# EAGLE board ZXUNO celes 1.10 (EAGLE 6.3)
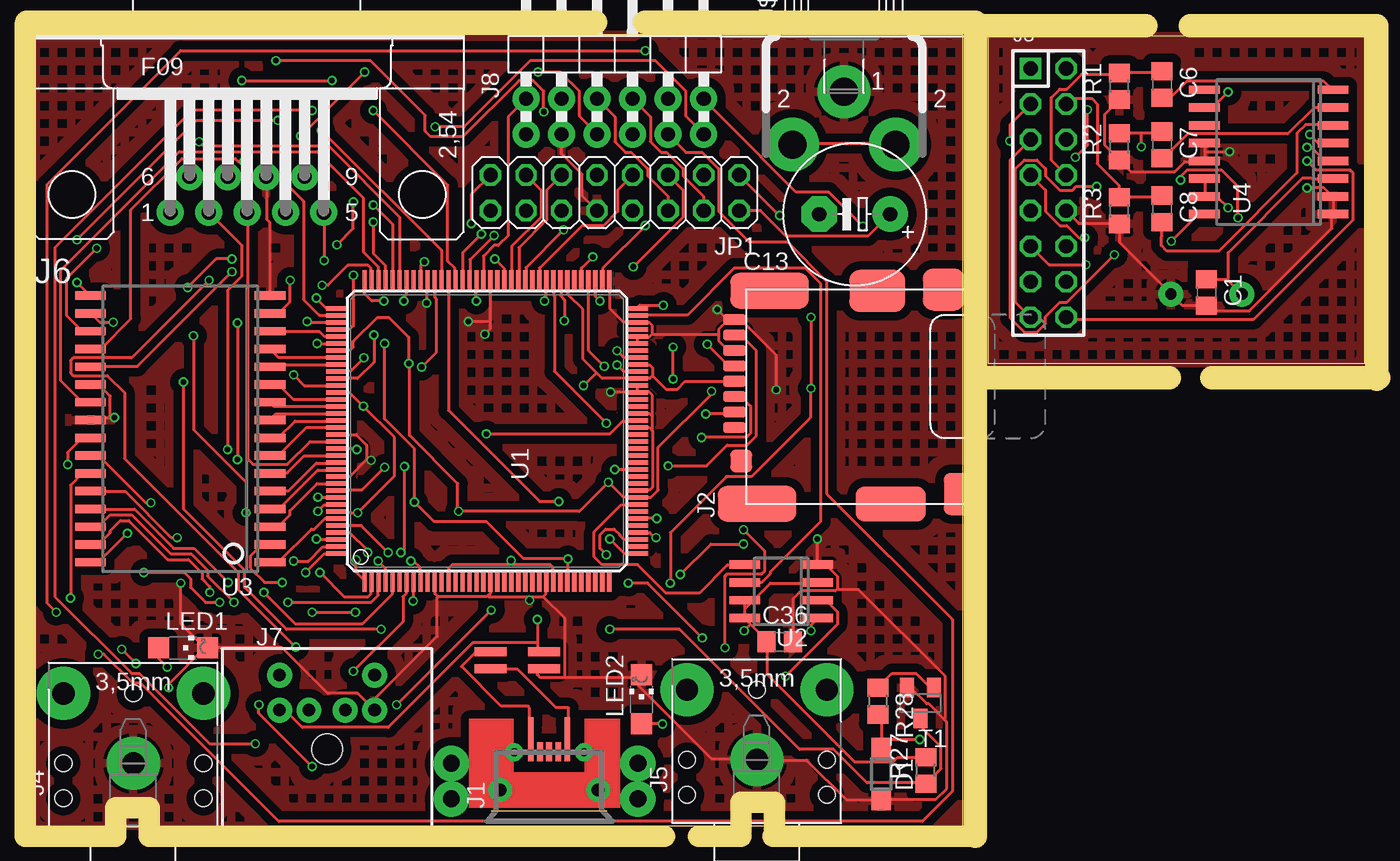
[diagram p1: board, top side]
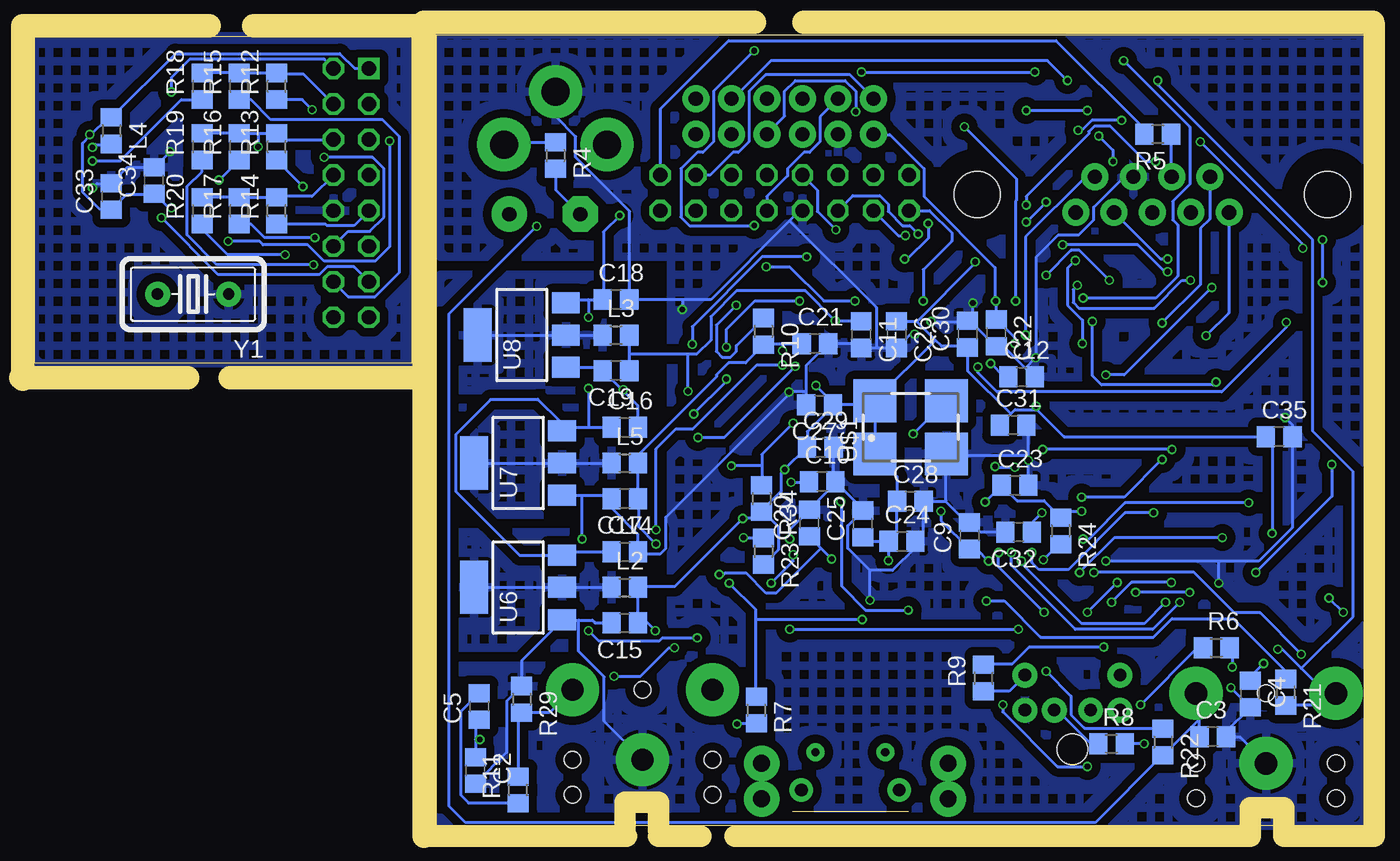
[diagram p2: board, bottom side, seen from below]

Size 95.05 x 56.49 mm. Coordinates in mm from the lower left corner, seen from the top.
Outline: 66.34,0 66.34,56.49 0,56.49 0,0 66.34,0
Outline: 68.12,56.39 68.12,33.02 95.05,33.02 95.05,56.39 68.12,56.39
Copper layers (1*16): Top 0.035mm / dielectric 1.5mm / Bottom 0.035mm
Design rules "default *": minimum track width 8mil, minimum drill 16mil, track to track 8mil, track to pad 8mil, pad to pad 8mil, via to via 10mil, smd to smd 8mil, copper to edge 0mil, drill to drill 10mil, minimum pad ring 5mil, minimum via ring 5mil, stop-mask expansion 4mil, vias tented up to drill 0mil, thermal gap 10mil
Net classes: 1 alimentacion: width 0.203 mm, drill 0.203 mm, clearance 0.203 mm
Milling: 19 lines

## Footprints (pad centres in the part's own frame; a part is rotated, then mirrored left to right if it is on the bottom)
C0805 = smd 1.3 x 1.5: 1 -0.95,0; 2 0.95,0
E5-10,5 = drill 1.016 pad 2.54: + -2.54,0 | drill 1.016 pad 2.54 octagon: - 2.54,0
SOD123 = smd 1.4 x 1.4: A 1.9,0; C -1.9,0
MICRO_USB = smd 1.35 x 0.4: 1 2.73,1.3; 2 2.73,0.65; 3 2.73,0; 4 2.73,-0.65; 5 2.73,-1.3; 6 4,1.3; 10 4,-1.3; 11 4.508,1.3; 13 4.508,-1.3 | drill 0.6 pad 1.27: P$1 2.7,2.5; P$2 2.7,-2.5 | drill 0.9 pad 1.676: P$3 0,3.5; P$4 0,-3.5 | drill 1.2 pad 2.54: P$5 -0.635,6.985; P$6 1.905,6.985; P$7 -0.635,-6.35; P$8 1.905,-6.35
MICRO_SD_CONNECTOR = smd 0.8 x 1.6: 1 -2.03,8.2; 2 -0.93,8.2; 3 0.17,8.2; 4 1.27,8.2; 5 2.37,8.2; 6 3.47,8.2; 7 4.57,8.2; 8 5.67,8.2 | smd 2.54 x 5.588: 9 7.735,5.7; 14 -7.49,6.6 | smd 3 x 4: 10 7.735,-2 | smd 3 x 3: 11 7.81,-6.75 | smd 3 x 2: 12 -6.79,-7.75 | smd 2.5 x 5: 13 -7.49,-2.95 | smd 1.6 x 1.55: 15 -4.43,7.725
DIL-100-2X08 = drill 1.016 square: 1 -8.89,-1.27 | drill 1.016 octagon: 2 -8.89,1.27; 3 -6.35,-1.27; 4 -6.35,1.27; 5 -3.81,-1.27; 6 -3.81,1.27; 7 -1.27,-1.27; 8 -1.27,1.27; 9 1.27,-1.27; 10 1.27,1.27; 11 3.81,-1.27; 12 3.81,1.27; 13 6.35,-1.27; 14 6.35,1.27; 15 8.89,-1.27; 16 8.89,1.27
STX = drill 1.6 pad 3.81: P$1 -0.762,-0.127; P$2 4.242,-5.131; P$3 4.242,4.877 | hole 1.2: -3.251,4.877; -0.762,4.877; -0.762,-5.131; -3.251,-5.131; 4.242,-0.127
F09H = drill 1.016 pad 1.93: 1 -5.486,-1.27; 2 -2.743,-1.27; 3 0,-1.27; 4 2.743,-1.27; 5 5.486,-1.27; 6 -4.115,1.27; 7 -1.372,1.27; 8 1.372,1.27; 9 4.115,1.27 | hole 3.302: -12.522,0; 12.522,0
MDIN06SS = drill 0.9 pad 1.778: 1 1.3,8.5; 2 -1.3,8.5; 3 3.4,8.5; 4 -3.4,8.5; 5 3.4,11; 6 -3.4,11 | hole 2.2: 0,5.716
2X06/90 = drill 1.016 pad 1.93: 1 -6.35,-6.35; 2 -6.35,-3.81; 3 -3.81,-6.35; 4 -3.81,-3.81; 5 -1.27,-6.35; 6 -1.27,-3.81; 7 1.27,-6.35; 8 1.27,-3.81; 9 3.81,-6.35; 10 3.81,-3.81; 11 6.35,-6.35; 12 6.35,-3.81
2X08 = drill 1.016 octagon: 1 -8.89,-1.27; 2 -8.89,1.27; 3 -6.35,-1.27; 4 -6.35,1.27; 5 -3.81,-1.27; 6 -3.81,1.27; 7 -1.27,-1.27; 8 -1.27,1.27; 9 1.27,-1.27; 10 1.27,1.27; 11 3.81,-1.27; 12 3.81,1.27; 13 6.35,-1.27; 14 6.35,1.27; 15 8.89,-1.27; 16 8.89,1.27
CHOKE_COMM = smd 1.27 x 0.635: P$1 -1.4,0.6; P$2 -1.4,-0.6; P$3 1.4,-0.6; P$4 1.4,0.6; P$5 -2.416,0.6; P$6 -2.416,-0.6; P$7 2.416,0.6; P$8 2.416,-0.6
0805 = smd 1.3 x 1.5: 1 -0.95,0; 2 0.95,0
CHIPLED_1206 = smd 1.5 x 1.5: A 0,-1.75; C 0,1.75
R0805 = smd 1.3 x 1.5: 1 -0.95,0; 2 0.95,0
SOT23 = smd 1 x 1.4: 1 -0.95,-1.1; 2 0.95,-1.1; 3 0,1.1
TQ144 = smd 1.6 x 0.3: P1 -10.7,8.75; P2 -10.7,8.25; P3 -10.7,7.75; P4 -10.7,7.25; P5 -10.7,6.75; P6 -10.7,6.25; P7 -10.7,5.75; P8 -10.7,5.25; P9 -10.7,4.75; P10 -10.7,4.25; P11 -10.7,3.75; P12 -10.7,3.25; P13 -10.7,2.75; P14 -10.7,2.25; P15 -10.7,1.75; P16 -10.7,1.25; P17 -10.7,0.75; P18 -10.7,0.25; P19 -10.7,-0.25; P20 -10.7,-0.75; P21 -10.7,-1.25; P22 -10.7,-1.75; P23 -10.7,-2.25; P24 -10.7,-2.75; P25 -10.7,-3.25; P26 -10.7,-3.75; P27 -10.7,-4.25; P28 -10.7,-4.75; P29 -10.7,-5.25; P30 -10.7,-5.75; P31 -10.7,-6.25; P32 -10.7,-6.75; P33 -10.7,-7.25; P34 -10.7,-7.75; P35 -10.7,-8.25; P36 -10.7,-8.75; P73 10.7,-8.75; P74 10.7,-8.25; P75 10.7,-7.75; P76 10.7,-7.25; P77 10.7,-6.75; P78 10.7,-6.25; P79 10.7,-5.75; P80 10.7,-5.25; P81 10.7,-4.75; P82 10.7,-4.25; P83 10.7,-3.75; P84 10.7,-3.25; P85 10.7,-2.75; P86 10.7,-2.25; P87 10.7,-1.75; P88 10.7,-1.25; P89 10.7,-0.75; P90 10.7,-0.25; P91 10.7,0.25; P92 10.7,0.75; P93 10.7,1.25; P94 10.7,1.75; P95 10.7,2.25; P96 10.7,2.75; P97 10.7,3.25; P98 10.7,3.75; P99 10.7,4.25; P100 10.7,4.75; P101 10.7,5.25; P102 10.7,5.75; P103 10.7,6.25; P104 10.7,6.75; P105 10.7,7.25; P106 10.7,7.75; P107 10.7,8.25; P108 10.7,8.75 | smd 0.3 x 1.6: P37 -8.75,-10.7; P38 -8.25,-10.7; P39 -7.75,-10.7; P40 -7.25,-10.7; P41 -6.75,-10.7; P42 -6.25,-10.7; P43 -5.75,-10.7; P44 -5.25,-10.7; P45 -4.75,-10.7; P46 -4.25,-10.7; P47 -3.75,-10.7; P48 -3.25,-10.7; P49 -2.75,-10.7; P50 -2.25,-10.7; P51 -1.75,-10.7; P52 -1.25,-10.7; P53 -0.75,-10.7; P54 -0.25,-10.7; P55 0.25,-10.7; P56 0.75,-10.7; P57 1.25,-10.7; P58 1.75,-10.7; P59 2.25,-10.7; P60 2.75,-10.7; P61 3.25,-10.7; P62 3.75,-10.7; P63 4.25,-10.7; P64 4.75,-10.7; P65 5.25,-10.7; P66 5.75,-10.7; P67 6.25,-10.7; P68 6.75,-10.7; P69 7.25,-10.7; P70 7.75,-10.7; P71 8.25,-10.7; P72 8.75,-10.7; P109 8.75,10.7; P110 8.25,10.7; P111 7.75,10.7; P112 7.25,10.7; P113 6.75,10.7; P114 6.25,10.7; P115 5.75,10.7; P116 5.25,10.7; P117 4.75,10.7; P118 4.25,10.7; P119 3.75,10.7; P120 3.25,10.7; P121 2.75,10.7; P122 2.25,10.7; P123 1.75,10.7; P124 1.25,10.7; P125 0.75,10.7; P126 0.25,10.7; P127 -0.25,10.7; P128 -0.75,10.7; P129 -1.25,10.7; P130 -1.75,10.7; P131 -2.25,10.7; P132 -2.75,10.7; P133 -3.25,10.7; P134 -3.75,10.7; P135 -4.25,10.7; P136 -4.75,10.7; P137 -5.25,10.7; P138 -5.75,10.7; P139 -6.25,10.7; P140 -6.75,10.7; P141 -7.25,10.7; P142 -7.75,10.7; P143 -8.25,10.7; P144 -8.75,10.7
SO-08 = smd 0.6 x 2.2: 1 -1.905,-2.6; 2 -0.635,-2.6; 3 0.635,-2.6; 4 1.905,-2.6; 5 1.905,2.6; 6 0.635,2.6; 7 -0.635,2.6; 8 -1.905,2.6
SOIC32 = smd 0.6 x 2.2: 1 -9.525,-6.416; 2 -8.255,-6.416; 3 -6.985,-6.416; 4 -5.715,-6.416; 5 -4.445,-6.416; 6 -3.175,-6.416; 7 -1.905,-6.416; 8 -0.635,-6.416; 9 0.635,-6.416; 10 1.905,-6.416; 11 3.175,-6.416; 12 4.445,-6.416; 13 5.715,-6.416; 14 6.985,-6.416; 15 8.255,-6.416; 16 9.525,-6.416; 17 9.525,6.416; 18 8.255,6.416; 19 6.985,6.416; 20 5.715,6.416; 21 4.445,6.416; 22 3.175,6.416; 23 1.905,6.416; 24 0.635,6.416; 25 -0.635,6.416; 26 -1.905,6.416; 27 -3.175,6.416; 28 -4.445,6.416; 29 -5.715,6.416; 30 -6.985,6.416; 31 -8.255,6.416; 32 -9.525,6.416
SO16W = smd 0.6 x 2.2: 1 -4.445,-4.6; 2 -3.175,-4.6; 3 -1.905,-4.6; 4 -0.635,-4.6; 5 0.635,-4.6; 6 1.905,-4.6; 7 3.175,-4.6; 8 4.445,-4.6; 9 4.445,4.6; 10 3.175,4.6; 11 1.905,4.6; 12 0.635,4.6; 13 -0.635,4.6; 14 -1.905,4.6; 15 -3.175,4.6; 16 -4.445,4.6
SOT223 = smd 1.5 x 2: 1 -2.3,-3.15; 2 0,-3.15; 3 2.3,-3.15 | smd 3.8 x 2: 4 0,3.15
SM77H = smd 3.048 x 3.048: 1 -2.55,-1.9; 2 2.55,-1.9; 3 2.55,1.9; 4 -2.55,1.9
RCA_PACK = drill 2 pad 3.81: 1 0,-3.945; 2 3.688,-7.72; 2@1 -3.688,-7.72
HC18U-V = drill 0.813 pad 1.778: 1 -2.54,0; 2 2.54,0

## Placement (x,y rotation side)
C1  8pF  [C0805]  83.74,38.1 270 top
C2  10nF  [C0805]  63.55,3.94 270 bottom
C3  10nF  [C0805]  10.85,6.35 0 bottom
C4  10nF  [C0805]  8.18,9.4 270 bottom
C5  100nF  [C0805]  63.3,8.51 90 bottom
C6  100nF  [C0805]  80.57,52.96 270 top
C7  100nF  [C0805]  80.57,48.64 270 top
C8  100nF  [C0805]  80.57,44.07 270 top
C9  100nF  [C0805]  28.24,20.71 90 bottom
C10  100nF  [C0805]  38.78,24.57 0 bottom
C11  100nF  [C0805]  35.98,35.08 270 bottom
C12  100nF  [C0805]  24.52,32.07 0 bottom
C13  220uF  [E5-10,5]  58.6,43.69 180 top
C14  1uF  [C0805]  52.88,19.56 0 bottom
C15  1uF  [C0805]  52.88,14.48 180 bottom
C16  1uF  [C0805]  52.88,28.45 0 bottom
C17  1uF  [C0805]  52.88,23.37 180 bottom
C18  1uF  [C0805]  53.52,37.59 0 bottom
C19  1uF  [C0805]  53.52,32.51 180 bottom
C20  100nF  [C0805]  39.68,21.62 90 bottom
C21  100nF  [C0805]  39.28,34.44 0 bottom
C22  100nF  [C0805]  26.33,35.21 270 bottom
C23  100nF  [C0805]  24.99,24.3 0 bottom
C24  100nF  [C0805]  33.06,20.31 0 bottom
C25  100nF  [C0805]  35.87,21.56 90 bottom
C26  100nF  [C0805]  33.46,35.08 270 bottom
C27  100nF  [C0805]  38.96,30.07 180 bottom
C28  100nF  [C0805]  32.46,23.18 0 bottom
C29  100nF  [C0805]  38.9,27.02 0 bottom
C30  100nF  [C0805]  28.38,35.12 90 bottom
C31  100nF  [C0805]  25.12,28.62 0 bottom
C32  100nF  [C0805]  24.73,20.96 180 bottom
C33  100nF  [C0805]  89.59,44.96 90 bottom
C34  10uF  [C0805]  86.54,46.1 90 bottom
C35  100nF  [C0805]  6.1,27.79 0 bottom
C36  100nF  [C0805]  53.24,13.13 0 top
D1  [SOD123]  60.5,3.68 270 top
J1  CON_MICRO_USB  [MICRO_USB]  36.75,2.54 90 top
J2  MICROSD_SPI_MODE  [MICRO_SD_CONNECTOR]  58.22,30.48 90 top
J3  J-16-100-2X08  [DIL-100-2X08]  72.44,45.21 270 top
J4  JACK_STEREO  [STX]  6.91,5.21 90 top
J5  JACK_STEREO  [STX]  51.49,5.46 90 top
J6  [F09H]  15.16,45.09 0 top
J7  [MDIN06SS]  20.88,-0.25 0 top
J8  JTAG_RGB  [2X06/90]  41.45,55.75 0 top
JP1  [2X08]  41.45,45.21 180 top
L1  BOBINA_VCC_ZXUNO  [CHOKE_COMM]  34.47,11.81 0 top
L2  FERRITE  [0805]  52.88,17.02 0 bottom
L3  FERRITE  [0805]  53.52,35.05 0 bottom
L4  FERRITE  [0805]  89.59,49.66 270 bottom
L5  FERRITE  [0805]  52.88,25.91 0 bottom
LED1  [CHIPLED_1206]  10.59,12.7 270 top
LED2  [CHIPLED_1206]  43.36,9.02 0 top
R1  75  [R0805]  77.52,52.83 90 top
R2  75  [R0805]  77.52,48.51 90 top
R3  75  [R0805]  77.52,43.94 90 top
R4  75  [R0805]  57.84,47.88 270 bottom
R5  270  [R0805]  14.78,49.4 180 bottom
R6  100  [R0805]  10.59,12.7 0 bottom
R7  220  [R0805]  43.48,8.26 270 bottom
R8  270  [R0805]  18.08,5.84 0 bottom
R9  270  [R0805]  27.23,10.54 90 bottom
R10  330  [R0805]  42.97,35.32 270 bottom
R11  470  [R0805]  60.5,2.54 90 bottom
R12  470  [R0805]  77.78,52.83 90 bottom
R13  470  [R0805]  77.78,48.51 90 bottom
R14  470  [R0805]  77.78,43.94 90 bottom
R15  1K  [R0805]  80.44,52.83 90 bottom
R16  1K  [R0805]  80.44,48.51 90 bottom
R17  1K  [R0805]  80.44,43.94 90 bottom
R18  2K  [R0805]  83.11,52.83 90 bottom
R19  2K  [R0805]  83.11,48.51 90 bottom
R20  2K  [R0805]  83.11,43.94 90 bottom
R21  3K9  [R0805]  5.64,9.53 270 bottom
R22  3K9  [R0805]  14.4,5.97 270 bottom
R23  4K7  [R0805]  42.97,19.6 270 bottom
R24  4K7  [R0805]  21.72,21.05 270 bottom
R27  1OK  [R0805]  63.68,3.94 90 top
R28  10K  [R0805]  60.25,8.89 270 top
R29  10K  [R0805]  60.25,9.02 270 bottom
R34  10K  [R0805]  43.1,23.37 270 bottom
T1  BC846  [SOT23]  63.3,8.76 180 top
U1  XC3S250ETQ144  [TQ144]  32.31,28.19 90 top
U2  W25X40BV  [SO-08]  53.35,16.74 90 top
U3  CY62148EV30  [SOIC32]  10.39,28.34 90 top
U4  AD724JR  [SO16W]  88.19,48.13 90 top
U6  LD117AS33TR  [SOT223]  60.5,17.02 90 bottom
U7  LD117AS25TR  [SOT223]  60.5,25.91 90 bottom
U8  LD117AS12TR  [SOT223]  60.25,35.05 90 bottom
U$1  SIT1602AC-83  [SM77H]  32.44,28.46 0 bottom
U$3  RCA_VIDEO  [RCA_PACK]  57.84,56.39 0 top
Y1  4.43M/3.58M  [HC18U-V]  83.74,37.97 180 bottom

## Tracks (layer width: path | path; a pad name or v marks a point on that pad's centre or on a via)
1.2V  (via drill 0.41)
  Top 0.203: v37.85,36.07 37.85,37.59 37.59,37.85 37.59,38.86 U1.P80 | U1.P115 21.64,33.98 22.55,33.98 22.76,34.19 22.76,34.59 24.49,36.32 25.3,36.32 26.72,34.9 v26.72,33.02 26.77,32.97 26.77,27.89 30.23,24.43 30.23,22.5 v30.28,22.45 38.91,22.45 v41,24.54 42.06,23.47 42.98,23.47 U1.P45 43.08,23.47 44.04,23.47 44.55,23.98 44.55,27.03 48.36,30.84 v48.36,31.04 | v26.87,18.9 27.08,18.9 27.53,18.44 27.53,17.53 U1.P9
  Bottom 0.203: 52.58,33.68 L3.2 | 52.58,33.68 C19.1 | C11.1 36.02,36.07 v37.85,36.07 39.98,38.2 44.91,38.2 46.74,36.37 46.74,34.7 47.75,33.68 48.36,33.68 | 48.36,33.68 52.58,33.68 | v26.72,33.02 25.81,32.11 25.5,32.11 C12.1 | v26.87,18.9 27.69,19.71 28.19,19.71 C9.1 28.3,19.81 30.28,21.79 v30.28,22.45 | v41,24.54 39.78,24.54 C10.1 | v48.36,31.04 48.36,33.68
2.5V  (via drill 0.41)
  Top 0.203: v26.36,37.49 26.36,37.8 26.52,37.95 26.52,38.86 U1.P102 | v41.61,33.93 42.06,33.48 42.98,33.48 U1.P65 | U1.P30 38.1,17.53 v38.1,19.05 38.05,19.1 34.9,19.1 32.26,21.74 28.5,21.74 v27.13,23.11 27.13,26.92 24.99,29.06 v24.99,34.44 | v20.22,22.45 20.68,22.91 21.59,22.91 U1.P137 | v50.65,20.12 48.31,20.12 v46.13,17.93
  Bottom 0.203: J8.1 35.1,49.38 33.94,49.38 31.5,46.94 31.5,44.96 26.42,39.88 26.42,37.54 v26.36,37.49 26.36,36.17 C22.1 26.26,36.12 24.99,34.85 v24.99,34.44 | 41.61,34.39 40.34,34.39 40.29,34.44 C21.1 | 41.61,34.39 42.93,34.39 R10.2 43.03,34.29 44.25,33.07 45.47,33.07 46.33,32.21 46.33,32.05 51.87,26.52 51.87,25.96 L5.2 51.97,25.91 51.97,23.37 C17.1 51.87,23.32 51.87,21.34 v50.65,20.12 | 41.61,34.39 v41.61,33.93 | v38.1,19.05 38.86,19.81 | 38.86,19.81 39.68,20.62 C20.1 | v20.22,22.45 22.05,22.45 R24.1 21.74,22.05 22.91,23.22 24.84,23.22 25.91,24.28 C23.1 26.01,24.23 v27.13,23.11 | v46.13,17.93 45.82,17.93 45.72,18.03 44.2,18.03 42.77,16.61 42.06,16.61 38.86,19.81
3.3V  (via drill 0.41)
  Top 0.203: U1.P138 21.64,22.4 22.55,22.4 22.61,22.35 v23.06,22.35 25.7,24.99 25.7,27.74 v23.47,29.97 22.5,30.94 21.64,30.94 U1.P121 | v27.84,40.28 27.58,40.03 27.58,38.91 U1.P100 | v6.6,20.88 4.57,18.85 4.01,18.85 U3.32 | 51.16,14.38 50.75,14.78 U2.8 50.75,14.88 50.75,15.54 | 51.16,14.38 52.27,13.26 52.27,13.16 C36.1 52.32,13.06 52.32,10.82 58.57,4.57 61.37,4.57 61.67,4.88 63.65,4.88 R27.2 | 50.75,15.54 50.75,16.05 U2.7 | U2.3 55.93,17.32 52.58,17.32 50.8,15.54 50.75,15.54 | 44.15,32.16 43.94,31.95 43.03,31.95 U1.P62 42.93,31.95 40.54,31.95 40.13,32.36 | 44.15,32.16 44.15,32.72 43.94,32.92 43.03,32.92 U1.P64 | 40.13,32.36 39.17,33.33 39.17,36.88 38.1,37.95 38.1,38.86 U1.P79 | J2.4 46.48,31.75 45.92,31.19 45.11,31.19 44.15,32.16 | v44.45,21.95 43.03,21.95 U1.P42 | 34.04,18.64 36.83,18.64 37.03,18.44 37.03,17.53 U1.P28 | 34.04,18.64 29.82,18.64 29.57,18.39 29.57,17.53 U1.P13 | v41.45,25.45 42.98,25.45 U1.P49 | v34.04,18.95 34.04,18.64 | v39.22,31.45 40.13,32.36 | v50.7,13.92 51.16,14.38
  Bottom 0.203: v23.06,22.35 23.77,21.64 23.77,20.98 C32.1 | 23.42,29.72 21.49,27.79 C35.1 6.96,27.74 6.6,27.38 v6.6,20.88 | 23.42,29.72 24.99,29.72 25.3,29.41 | 25.3,29.41 26.06,28.65 C31.1 | 25.3,29.41 28.35,32.46 28.35,34.14 C30.1 28.45,34.24 30.23,34.24 30.68,34.7 | 32,36.02 33.43,36.02 C26.1 | 30.68,34.7 32,36.02 | v27.84,40.28 27.84,40.18 32,36.02 | v23.47,29.97 23.47,29.77 23.42,29.72 | R23.2 42.93,18.69 41.91,19.71 41.91,21.34 42.98,22.4 43.08,22.4 R34.2 | R34.2 42.62,21.95 v44.45,21.95 49.33,17.07 51.87,17.07 L2.2 51.97,17.02 51.97,14.48 C15.1 51.92,15.14 v50.7,13.92 | C24.1 34.04,20.32 35.61,20.32 35.87,20.57 C25.1 | C24.1 33.94,20.37 33.43,20.88 33.43,23.16 C28.1 33.43,23.27 33.43,24.94 34.95,26.47 U$1.1 35,30.23 U$1.4 | C27.1 38,30.07 35.26,30.07 35,30.33 U$1.4 | C27.1 38,29.97 39.83,28.14 39.83,27.03 C29.1 39.93,26.98 v41.45,25.45 41.71,25.2 41.71,23.88 42.93,22.66 42.93,22.45 R34.2 | v34.04,18.95 34.04,20.22 C24.1 | v39.22,31.45 37.9,30.12 C27.1 | 30.68,34.7 34.95,30.43 U$1.4
5V  (via drill 0.41)
  Top 0.203: JP1.1 v53.24,43.59 | v55.47,36.32 v55.47,31.24 55.42,31.19 55.42,29.16 51.21,24.94 49.43,24.94 45.41,20.93 v45.41,17.32 | v35.92,14.73 35.92,13.06 | 35.92,13.06 35.92,12.45 L1.P$4 | J7.4 17.53,8.23 17.88,8.23 19.1,7.01 25.25,7.01 31.29,13.06 35.92,13.06
  Bottom 0.203: C14.1 57.1,19.56 57.3,19.36 U6.3 57.46,19.3 60.4,19.3 64.97,23.88 64.97,27.94 62.48,30.43 59.18,30.43 59.11,30.48 57.46,28.83 57.46,28.19 U7.3 57.3,28.25 57.1,28.45 55.47,28.45 | 55.47,28.45 C16.1 | 55.47,37.59 56.84,37.59 57.05,37.39 U8.3 | 55.47,37.59 C18.1 54.41,37.64 54.41,42.42 v53.24,43.59 | JP1.1 50.34,51.21 45.47,56.08 22.05,56.08 15.75,49.78 15.75,49.43 R5.2 | v55.47,31.24 55.47,28.45 | 55.47,37.59 v55.47,36.32 | 43.54,14.73 43.54,15.44 v45.41,17.32 | 43.54,14.73 43.54,9.3 R7.1 | 43.54,14.73 v35.92,14.73
5V_  (via drill 0.41)
  Top 0.203: U4.14 83.62,46.23 83.62,44.96 U4.15 83.67,44.91 84.53,44.91 v85.29,44.15 | U4.5 91.75,48.77 v91.14,49.38
  Bottom 0.203: 91.09,49.33 91.64,48.77 91.64,45.26 90.42,44.04 89.66,44.04 C33.1 89.56,44.04 88.49,45.11 86.56,45.11 C34.1 86.46,45.11 85.5,44.15 v85.29,44.15 | 91.09,49.33 89.81,50.6 89.61,50.6 L4.1 89.51,50.65 84.99,55.17 73.25,55.17 72.19,54.1 J3.1 | v91.14,49.38 91.09,49.33
B
  Top 0.203: JP1.4 47.8,44.96 46.33,46.43 46.33,46.94 45.16,48.11 44.76,48.11 43.99,48.87 43.99,50.65 42.72,51.92 J8.8
B0  (via drill 0.41)
  Top 0.203: v31.55,37.49 31.55,38.86 U1.P92
  Bottom 0.203: v31.55,37.49 31.55,39.73 29.51,41.76 29.51,42.37 31.09,43.94 JP1.16
B0_  (via drill 0.41)
  Top 0.203: v90.93,47.5 91.59,46.84 94.03,46.84 94.23,46.63 94.23,43.28 87.12,36.17 73.86,36.17 J3.16
  Bottom 0.203: v90.93,47.5 88.95,47.5 84.58,51.87 83.11,51.87 R18.1
B1  (via drill 0.41)
  Top 0.203: v32.82,42.16 31.09,40.44 31.09,38.91 U1.P93
  Bottom 0.203: v32.82,42.16 33.33,42.16 JP1.14
B1_
  Bottom 0.203: J3.14 72.64,37.8 70.71,37.8 68.99,39.52 68.99,49.23 70.21,50.44 78.18,50.44 79.6,51.87 80.42,51.87 R15.1
B2  (via drill 0.41)
  Top 0.203: v31.9,42.27 30.58,40.95 30.58,38.91 U1.P94
  Bottom 0.203: v31.9,42.27 32.51,42.88 33.02,42.88 34.04,43.89 34.04,44.4 34.65,45.01 36.58,45.01 JP1.12
B2_  (via drill 0.41)
  Top 0.203: v75.23,51.16 75.23,48.62 v74.37,47.75
  Bottom 0.203: v75.23,51.16 75.95,51.87 77.78,51.87 R12.1 | v74.37,47.75 70.92,47.75 70.1,46.94 70.1,43.48 71.12,42.47 72.64,42.47 J3.12
B_
  Top 0.203: C8.1 80.47,44.91 77.52,44.91 R3.2 77.47,44.96 77.47,45.77 75.95,47.3 75.95,51.56 75.54,51.97 74.12,51.97 J3.4
  Bottom 0.203: R18.2 83.11,53.8 80.52,53.8 R15.2 80.42,53.8 77.78,53.8 R12.2 77.72,53.7 75.84,53.7 J3.4
CLK  (via drill 0.41)
  Top 0.203: v32.26,27.99 41.1,27.99 42.01,28.91 42.98,28.91 U1.P56
  Bottom 0.203: v32.26,27.99 29.92,30.33 U$1.3
CMPS
  Top 0.203: JP1.2 51.87,43.94 53.7,42.11 59.54,42.11 61.11,43.69 C13.+
CMPS_  (via drill 0.41)
  Top 0.203: U4.10 84.18,51.31 v85.29,52.43
  Bottom 0.203: v85.29,52.43 85.29,53.44 83.97,54.76 74.37,54.76 J3.2
CSYNC
  Top 0.203: U1.P91 32.05,38.91 32.05,40.69 32.82,41.45 33.12,41.45 33.83,42.16 33.83,50.65 35.1,51.92 J8.2
  Bottom 0.203: JP1.3 46.79,46.48 45.16,48.11 44.76,48.11 43.99,48.87 43.99,52.48 42.83,53.65 36.78,53.65 35.1,51.97 J8.2
CSYNC_  (via drill 0.41)
  Top 0.203: U4.16 83.16,43.69 v81.23,41.76 | v69.7,48.92 69.7,50.09 J3.3
  Bottom 0.203: v81.23,41.76 78.99,41.76 78.74,41.5 75.54,41.5 74.37,40.34 70.71,40.34 69.7,41.35 v69.7,48.92
EAR  (via drill 0.41)
  Top 0.203: T1.3 63.3,7.11 64.77,5.64 64.77,4.06 63.7,3 R27.1 63.6,3.05 59.49,3.05 57.1,5.44 54.66,5.44 46.08,14.02 v41.1,14.02 | v19.46,36.02 19.51,35.97 21.59,35.97 U1.P111 | v10.62,31.7 10.62,22.61 14.99,18.24 14.99,17.02 17.98,14.02 v24.74,14.02
  Bottom 0.203: v19.46,36.02 19.46,32.16 18.8,31.5 10.82,31.5 v10.62,31.7 | v41.1,14.02 v24.74,14.02
FLASH_CS  (via drill 0.41)
  Top 0.203: v40.84,19.36 40.39,19.81 40.39,20.78 40.79,21.18 41.4,21.18 41.81,20.78 41.81,20.73 42.06,20.47 42.98,20.47 U1.P39 | v42.42,17.32 43.79,17.32 v47.7,13.41 | v55.47,13.92 55.47,14.33 55.93,14.78 U2.1
  Bottom 0.203: v40.84,19.36 40.84,18.9 v42.42,17.32 | v47.7,13.41 50.19,13.41 50.39,13.21 54.76,13.21 v55.47,13.92
FLASH_MISO  (via drill 0.41)
  Top 0.203: v41.61,32.92 42.06,32.46 42.98,32.46 U1.P63 | v50.65,21.13 52.17,19.61 52.17,18.19 51.97,17.98 49.48,17.98 49.33,17.83 v49.33,12.7 | v53.65,10.67 57.35,14.38 57.35,15.29 56.59,16.05 55.98,16.05 U2.2
  Bottom 0.203: v41.61,32.92 43.43,32.92 48.01,28.35 49.23,28.35 50.65,26.92 v50.65,21.13 | v49.33,12.7 49.73,12.7 51.77,10.67 v53.65,10.67
FLASH_MOSI
  Top 0.203: U1.P44 42.98,22.91 41.91,22.91 39.98,20.98 39.98,19.2 40.54,18.64 43.08,18.64 45.11,16.61 47.5,16.61 49.48,18.59 50.7,18.59 U2.5
FLASH_SCK
  Top 0.203: U1.P71 43.03,36.47 46.64,36.47 49.99,39.83 55.07,39.83 56.19,38.71 56.19,21.74 52.58,18.14 52.58,17.98 51.97,17.37 U2.6
G
  Top 0.203: JP1.6 45.26,44.96 43.79,46.43 43.79,46.94 42.62,48.11 42.22,48.11 41.45,48.87 41.45,50.65 40.18,51.92 J8.6
G0
  Top 0.203: JP1.11 36.58,45.41 36.58,43.28 34.59,41.3 34.59,38.91 U1.P86
G0_  (via drill 0.41)
  Top 0.203: v75.13,40.08 72.49,40.08 J3.11
  Bottom 0.203: R19.1 83.11,46.74 84.18,45.67 84.18,42.22 82.04,40.08 v75.13,40.08
G1
  Top 0.203: JP1.13 36.17,45.41 36.17,43.48 34.09,41.4 34.09,38.91 U1.P87
G1_  (via drill 0.41)
  Top 0.203: v81.89,46.13 81.89,46.38 82.35,46.84 84.84,46.84 86,45.67 v86,43.43
  Bottom 0.203: v81.89,46.13 80.47,47.55 R16.1 | v86,43.43 81.94,39.37 74.73,39.37 74.17,39.93 72.24,39.93 J3.13
G2  (via drill 0.41)
  Top 0.203: v32.87,40.49 33.53,39.83 33.53,38.91 U1.P88 | v31.19,43.03 31.19,45.11 JP1.15
  Bottom 0.203: v32.87,40.49 32.66,40.49 31.19,41.96 v31.19,43.03
G2_  (via drill 0.41)
  Top 0.203: v75.89,45.67 74.42,45.67 74.17,45.41 73.25,45.41 72.24,46.43 72.24,46.94 71.63,47.55 70.71,47.55 70.1,46.94 70.1,37.39 J3.15
  Bottom 0.203: v75.89,45.67 77.78,47.55 R13.1
G_  (via drill 0.41)
  Top 0.203: 79.1,49.48 80.47,49.48 C7.1 | 79.1,49.48 77.52,49.48 R2.2 | v79.1,48.51 79.1,49.48
  Bottom 0.203: 79.1,49.48 80.42,49.48 R16.2 80.52,49.48 83.11,49.48 R19.2 | 79.1,49.48 77.78,49.48 R13.2 77.72,49.38 77.37,49.02 J3.6 | 79.1,49.48 v79.1,48.51
GND  (via drill 0.41)
  Top 0.203: U3.16 16.76,37.9 16.76,43.13 16.56,43.33 16.56,46.33 J6.8 | v23.52,33.43 22.55,32.46 21.64,32.46 U1.P118 | v27.99,37.34 28.04,37.39 28.04,38.86 U1.P99 | U1.P60 43.03,30.99 43.03,31.39 U1.P61 | 44.09,28.25 43.89,28.45 43.03,28.45 U1.P55 | 44.09,28.25 44.15,28.19 44.15,24.18 43.94,23.98 43.03,23.98 U1.P46 | 44.09,29.26 44.15,29.21 44.15,28.3 44.09,28.25 | 44.09,29.26 43.94,29.41 43.03,29.41 U1.P57 | U1.P60 43.13,30.99 43.89,30.99 44.15,30.73 44.15,29.31 44.09,29.26 | 32.56,36.02 32.56,35.51 v32.16,35.1 | 32.56,36.02 32.56,38.86 U1.P90 | v41.15,30.99 42.93,30.99 U1.P60 | 32.56,36.02 v30.99,36.02 | 48.87,35.1 48.87,35.46 49.53,36.12 49.99,36.12 J2.8 | 48.87,35.1 48.87,34.65 49.53,33.98 49.99,33.98 J2.6 | U1.P67 43.03,34.49 43.03,34.9 U1.P68 43.13,34.9 43.89,34.9 44.15,35.15 | 44.15,35.15 44.15,35.71 43.94,35.92 43.03,35.92 U1.P70 42.93,35.97 42.06,35.97 41.1,36.93 41.1,38.86 U1.P73 | 48.87,35.1 44.2,35.1 44.15,35.15 | v52.98,31.14 52.98,33.63 50.5,36.12 50.09,36.12 J2.8 | J8.3 37.64,48.01 39.12,46.53 39.12,45.01 JP1.10 | v48.77,36.88 49.48,36.17 J2.8 | 57.35,16.92 57.2,16.76 54.76,16.76 54.2,16.2 54.2,13.16 C36.2 | 57.35,16.92 57.35,17.83 56.59,18.59 55.98,18.59 U2.4 | U2.4 | 65.02,7.57 65.18,7.42 65.18,2.64 64.42,1.88 60.55,1.88 D1.A 60.5,1.83 58.01,1.83 55.17,4.67 51.61,4.67 J5.P$1 51.56,4.78 48.36,4.78 42.62,10.52 LED2.C 43.33,10.72 43.18,10.57 37.85,10.57 | 65.02,7.57 63.91,8.69 63.75,8.69 62.59,9.86 62.38,9.86 T1.2 | 57.35,16.92 57.4,16.87 58.88,16.87 65.08,10.67 65.08,7.62 65.02,7.57 | v55.93,20.47 55.93,18.75 U2.4 | v41.1,20.47 42.11,19.46 42.98,19.46 U1.P37
  Top 0.203: 23.72,26.16 22.5,24.94 21.64,24.94 U1.P133 | 23.72,26.16 23.72,27.18 22.96,27.94 21.64,27.94 U1.P127 | v24.03,26.11 23.77,26.11 23.72,26.16 | U3.24 4.01,29.01 4.17,29.16 v5.69,29.16 5.38,29.21 5.38,30.68 4.57,31.5 4.01,31.5 U3.22 | v18.49,18.9 19.56,18.9 20.57,19.91 21.59,19.91 U1.P143 | 37.85,10.57 36.12,10.57 35.92,10.77 35.92,11.18 L1.P$3 | 28.8,16.36 28.6,16.56 28.6,17.48 U1.P11 | 28.8,16.36 32.31,16.36 32.36,16.41 | 32.36,16.41 32.56,16.61 32.56,17.48 U1.P19 | 36.32,16.36 36.52,16.56 36.52,17.48 U1.P27 | 35.36,16.36 32.41,16.36 32.36,16.41 | 35.36,16.36 36.32,16.36 | 37.85,10.57 37.85,14.83 36.32,16.36 | LED1.C 17.68,12.7 20.93,9.45 23.06,9.45 24.23,8.28 J7.3 23.93,8.69 28.75,13.51 28.75,16.31 28.8,16.36 | v9.55,9.86 9.55,10.11 12.14,12.7 LED1.C | v10.41,17.32 10.41,14.43 12.09,12.75 LED1.C | 35.36,16.36 v35.36,16.1
  Bottom 0.203: 24.26,32.69 25.81,34.24 26.31,34.24 C22.2 26.42,34.29 28.14,36.02 28.35,36.02 C30.2 | 24.26,32.69 23.67,32.11 23.57,32.11 C12.2 | 24.26,32.69 v23.52,33.43 23.47,33.48 23.47,40.64 21.89,42.22 20.42,42.22 19.35,43.28 19.35,44.2 17.22,46.33 16.56,46.33 J6.8 | v27.99,37.34 27.99,35.97 C30.2 | 34.9,34.14 35.97,34.14 C11.2 36.07,34.19 36.32,34.44 38.3,34.44 C21.2 38.41,34.39 39.93,32.87 39.93,30.99 | 34.9,34.14 33.48,34.14 C26.2 33.38,34.19 32.46,35.1 v32.16,35.1 | 39.93,30.99 39.93,30.07 C27.2 | 39.93,30.99 v41.15,30.99 41.2,30.94 41.2,30.79 49.94,22.05 49.94,19.81 50.34,19.41 51.77,19.41 51.87,19.51 C14.2 51.97,19.56 51.97,20.83 53.8,22.66 53.8,23.37 C17.2 53.9,23.42 54.05,23.57 55.93,23.57 | v30.99,36.02 28.45,36.02 C30.2 | 53.04,31.09 54.46,32.51 C19.2 54.56,32.56 54.71,32.72 57.05,32.72 U8.1 | 53.04,31.09 51.97,30.02 51.97,28.45 C16.2 | v52.98,31.14 53.04,31.09 | 48.77,37.59 46.74,37.59 41.1,43.23 | 48.77,37.59 C18.2 52.53,37.64 52.53,43.89 56.39,47.75 56.39,49.23 57.81,50.65 57.81,52.43 U$3.1 | 41.1,43.23 40.39,43.94 JP1.10 | 48.77,37.59 v48.77,36.88 | 34.9,34.14 34.9,37.03 41.1,43.23 | C2.2 61.32,5.23 61.32,8.89 60.3,9.91 R29.1 60.25,11.79 57.35,14.68 U6.1 57.25,14.68 56.19,14.68 | C15.2 55.02,14.48 55.22,14.68 56.19,14.68 | 55.93,23.57 57.3,23.57 U7.1 | v55.93,20.47 55.93,23.57 | 56.19,14.68 56.19,12.45 54.36,10.62 54.36,7.47 51.61,4.72 J5.P$1 | C10.2 37.8,24.54 35.92,22.66 35.92,22.55 C25.2 35.92,22.45 36.93,21.44 36.93,19.81 35.36,18.24 | C29.2 37.95,26.98 37.95,24.69 37.9,24.64 C10.2 | C10.2 37.8,24.49 39.68,22.61 C20.2 39.73,22.5 41.1,21.13 v41.1,20.47
  Bottom 0.203: 24.08,26.47 24.08,28.55 24.13,28.6 C31.2 | 24.08,26.47 24.08,26.11 | 24.08,26.11 24.08,24.33 C23.2 | v24.03,26.11 24.08,26.11 | 29.92,26.57 U$1.2 | C32.2 25.7,20.98 27.53,20.98 28.19,21.64 C9.2 28.3,21.74 28.55,21.74 29.97,23.16 | 29.97,23.16 31.44,23.16 C28.2 31.55,23.16 31.55,20.88 C24.2 32.11,20.22 32.11,19.86 33.73,18.24 35.36,18.24 | U$1.2 29.92,26.47 29.92,23.22 29.97,23.16 | 24.08,26.47 29.82,26.47 U$1.2 | v5.69,29.16 5.18,28.65 5.18,27.79 C35.2 5.18,27.69 5.18,21.29 7.57,18.9 10.41,18.9 | 10.41,18.9 v18.49,18.9 | J4.P$1 8.89,6.3 9.8,6.3 C3.2 9.86,6.35 9.86,6.76 8.18,8.43 C4.2 8.23,8.53 v9.55,9.86 | v10.41,17.32 10.41,18.9 | v35.36,16.1 35.36,18.24
  pour Bottom (isolate 0.61, hatched): 0.05,56.52 0.05,0 66.09,0 66.09,11.43 49.58,11.43 49.58,40.64 66.09,40.64 66.09,56.52
  pour Top (isolate 0.61, hatched): 0.05,56.52 0.05,0 66.09,0 66.09,56.52
GND_  (via drill 0.41)
  Top 0.203: 83.62,48.16 83.62,48.77 U4.12 | 83.62,48.16 83.62,47.5 U4.13 83.52,47.45 82.2,47.45 81.48,46.74 78.33,46.74 77.57,47.5 R2.1 77.52,47.6 76.45,48.67 76.45,50.8 77.52,51.87 R1.1 | 83.62,48.16 v85.39,48.16 | J3.10 74.62,43.03 77.52,43.03 R3.1 77.57,42.93 77.57,41.66 81.18,38.05 Y1.1 81.99,37.19 83.72,37.19 C1.2 83.82,37.08 84.12,36.78 86.82,36.78 92.71,42.67 92.71,43.64 U4.1 92.81,43.69 92.81,44.96 U4.2 92.71,45.01 92.15,45.57 v90.93,45.57
  Bottom 0.203: v85.39,48.16 86.46,47.09 C34.2 86.56,47.04 88.44,47.04 89.56,45.92 C33.2 89.66,45.87 90.63,45.87 v90.93,45.57
  pour Top (isolate 0.61, hatched): 68.12,56.39 94.79,56.39 94.79,33.02 68.12,33.02
  pour Bottom (isolate 0.61, hatched): 68.12,56.39 95.05,56.39 95.05,33.02 68.12,33.02
JOY1  (via drill 0.41)
  Top 0.203: v23.77,19.51 23.77,19.66 22.5,20.93 21.64,20.93 U1.P141 | v15.09,22.35 15.09,24.54 11.33,28.3 v11.33,35
  Bottom 0.203: v23.77,19.51 23.77,18.8 23.27,18.29 21.18,18.29 17.12,22.35 v15.09,22.35 | v11.33,35 9.7,36.63 9.7,43.79 J6.1
JOY2  (via drill 0.41)
  Top 0.203: v23.01,26.87 22.96,26.92 21.64,26.92 U1.P129 | v13.77,26.87 13.77,38.25 14.78,39.27 14.78,41.45 J6.2
  Bottom 0.203: v13.77,26.87 v23.01,26.87
JOY3
  Top 0.203: U1.P128 21.59,27.43 19.66,27.43 18.03,25.81 15.6,25.81 15.19,26.21 15.19,43.79 J6.3
JOY4  (via drill 0.41)
  Top 0.203: v18.49,32.21 19.25,31.45 21.59,31.45 U1.P120 | v10.92,38.46 12.95,40.49 v14.07,40.49
  Bottom 0.203: v18.49,32.21 17.17,32.21 v10.92,38.46 | v14.07,40.49 14.58,40.49 J6.4
JOY5  (via drill 0.41)
  Top 0.203: v20.22,23.47 21.59,23.47 U1.P136 | v14.48,35.92 v14.48,26.16
  Bottom 0.203: v20.22,23.47 17.17,23.47 v14.48,26.16 | v14.48,35.92 11.73,38.66 11.73,42.67 11.07,43.33 11.07,46.33 J6.6
JOY6  (via drill 0.41)
  Top 0.203: v20.17,34.44 21.59,34.44 U1.P114 | v20.68,40.39 20.68,43.79 J6.5
  Bottom 0.203: v20.17,34.44 20.17,36.12 21.23,37.19 21.23,39.83 v20.68,40.39
JOY7  (via drill 0.41)
  Top 0.203: v24.23,35.05 24.23,33.12 23.06,31.95 21.64,31.95 U1.P119
  Bottom 0.203: v24.23,35.05 24.23,42.06 19.96,46.33 19.3,46.33 J6.9
L-OUT  (via drill 0.41)
  Top 0.203: v59.18,42.82 56.74,45.26 54.41,45.26 51.92,47.75 51.92,47.8 47.8,51.92 J8.12
  Bottom 0.203: 11.84,7.52 11.84,9.25 J4.P$2 | 11.84,7.52 11.84,6.35 C3.1 | 11.84,7.52 11.89,7.52 14.38,5.03 R22.2 14.48,4.98 19.25,0.2 64.26,0.2 65.43,1.37 65.43,36.58 v59.18,42.82
LED  (via drill 0.41)
  Top 0.203: v16,8.64 16,8.03 v19.81,4.22 | v37.44,23.16 36.07,23.16 29.57,29.67 29.57,38.86 U1.P96 | v32.61,15.39 v25.86,8.64
  Bottom 0.203: R6.1 11.94,12.7 v16,8.64 | v19.81,4.22 21.95,4.22 25.86,8.13 v25.86,8.64 | v32.61,15.39 35.66,15.39 37.39,17.12 37.39,23.11 v37.44,23.16
LEFT  (via drill 0.41)
  Top 0.203: v22.76,11.02 26.31,14.58 26.31,16.36 26.52,16.56 26.52,17.48 U1.P7
  Bottom 0.203: v22.76,11.02 20.98,9.25 20.98,7.92 20.01,6.96 14.43,6.96 R22.1
N$1
  Top 0.203: C8.2 80.57,42.11 80.52,42.06 80.52,41.45 80.92,41.05 84.63,41.05 90.22,46.63 90.22,49.48 90.83,50.09 92.71,50.09 92.76,50.04 U4.6
N$2
  Top 0.203: U4.7 91.44,51.31 89.56,49.43 82.4,49.43 80.67,47.7 80.57,47.7 C7.2
N$3
  Top 0.203: C6.2 81.18,52.02 82.35,53.19 92.15,53.19 92.76,52.58 U4.8
N$5  (via drill 0.41)
  Top 0.203: v9.45,11.33 8.89,11.89 8.89,12.7 LED1.A
  Bottom 0.203: v9.45,11.33 9.45,12.55 9.6,12.7 R6.2
N$6
  Top 0.203: 85.24,39.01 83.77,39.01 C1.1 | Y1.2 85.24,39.01 | U4.3 91.29,46.23 91.24,46.28 90.63,46.28 85.29,40.95 85.29,39.06 85.24,39.01
N$8  (via drill 0.41)
  Top 0.203: v44.86,7.26 43.38,7.26 LED2.A
  Bottom 0.203: v44.86,7.26 43.48,7.26 R7.2
N$9
  Bottom 0.203: R4.2 57.81,46.89 57.81,45.41 56.08,43.69 C13.-
N$10
  Top 0.203: U$3.2@1 54.15,48.72 61.52,48.72 U$3.2
  Bottom 0.203: R4.1 57.86,48.82 61.42,48.82 61.52,48.72 U$3.2
N$11
  Top 0.203: T1.1 64.21,9.91 63.96,9.91 62.99,10.87 61.27,10.87 60.25,9.86 R28.1
N$12  (via drill 0.41)
  Top 0.203: R28.2 60.25,7.92 60.5,7.67 D1.C 60.55,6.15 v63.25,6.15
  Bottom 0.203: 63.55,6.15 63.55,7.26 63.3,7.52 C5.1 | 63.55,6.15 C2.1 | 63.55,6.15 v63.25,6.15
N$13
  Bottom 0.203: R11.1 60.5,1.63 64.06,1.63 64.62,2.18 64.62,8.13 C5.2
N$14
  Bottom 0.203: J5.P$2 56.64,9.7 58.27,8.08 R29.2 60.3,7.98 60.5,7.77 R11.2
N$15  (via drill 0.41)
  Top 0.203: v22.96,19 22.96,18.09 23.52,17.53 U1.P1
  Bottom 0.203: v22.96,19 21.89,20.07 21.74,20.07 R24.2
N$16  (via drill 0.41)
  Top 0.203: v44.91,37.19 43.23,37.19 43.03,36.98 U1.P72
  Bottom 0.203: v44.91,37.19 46.33,35.76 46.33,33.88 45.92,33.48 45.31,33.48 44.91,33.88 44.91,34.29 42.98,36.22 R10.1
N$17  (via drill 0.41)
  Top 0.203: v44.4,20.57 44.3,20.57 43.94,20.93 43.03,20.93 U1.P40
  Bottom 0.203: v44.4,20.57 42.98,20.57 R23.1
N$18
  Bottom 0.203: R8.1 19.56,5.84 21.95,8.23 22.15,8.23 J7.1
N$19
  Bottom 0.203: R9.1 27.23,9.6 25.4,9.6 24.28,10.72 J7.5
N$20
  Bottom 0.203: R5.1 13.82,49.38 13.82,46.38 J6.7
N$21
  Bottom 0.203: U6.2 L2.1 | U6.4 U6.2 | 57.46,16.97 U6.2 | U6.2 | U6.2 57.42,16.95
  pour Bottom (isolate 0.61, hatched): 51.49,20.95 66.09,20.95 66.09,12.7 51.49,12.7
N$22
  Bottom 0.203: L5.1 U7.2 U7.4
  pour Bottom (isolate 0.61, hatched): 52.76,29.84 66.09,29.84 66.09,22.23 52.76,22.23
N$23
  Bottom 0.203: L3.1 U8.2 U8.4
  pour Bottom (isolate 0.61, hatched): 53.39,39.37 66.09,39.37 66.09,31.11 53.39,31.11
N$24  (via drill 0.41)
  Top 0.203: v90.93,48.46 91.24,48.46 92.2,47.5 U4.4
  Bottom 0.203: v90.93,48.46 90.73,48.67 89.61,48.67 L4.2
N$25
  Top 0.203: 35.36,5.27 35.36,8.38 35.26,8.53 33.33,8.53 30.48,11.38 31.44,12.34 | 33.27,12.39 33.17,12.39 | 33.17,12.39 33.07,12.39 | 33.17,12.39 L1.P$1 | 33.33,12.34 L1.P$1 | 33.43,12.34 L1.P$1
  Top 0.254: 31.55,12.45 33.03,12.45 L1.P$1 | 33.43,12.34 31.44,12.34
  Top 0.406: J1.1 35.36,5.27
N$26
  Top 0.203: 38.15,5.27 38.15,8.38 38.1,8.43 37.24,8.43 34.49,11.18 33.27,11.18 L1.P$2 | 33.07,11.18 L1.P$2 | 33.17,11.18 L1.P$2
  Top 0.406: J1.5 38.15,5.27
PS2_CLK  (via drill 0.41)
  Top 0.203: v18.64,12.75 14.53,16.87 14.53,18.09 6.4,26.21 6.4,30.94 5.18,32.16 2.74,32.16 2.54,32.36 2.54,33.22 2.74,33.43 6.91,33.43 v12.45,38.96 | v20.52,38.61 20.93,38.61 22.35,40.03 23.82,40.03 24.03,39.83 24.03,38.91 U1.P107
  Bottom 0.203: v18.64,12.75 23.98,12.75 25.2,11.53 27.23,11.53 R9.2 | v12.45,38.96 13.06,38.96 15.04,36.98 20.42,36.98 20.83,37.39 20.83,38.3 v20.52,38.61
PS2_DATA  (via drill 0.41)
  Top 0.203: v15.75,5.84 12.5,5.84 7.47,10.87 6.91,10.87 1.42,16.36 1.42,41.3 11.23,51.1 v19.81,51.1 | v24.18,51.1 29.51,45.77 29.51,40.34 30.02,39.83 30.02,38.91 U1.P95
  Bottom 0.203: v15.75,5.84 R8.2 | v24.18,51.1 v19.81,51.1
R
  Bottom 0.203: JP1.8 42.72,44.96 41.25,46.43 41.25,46.94 40.08,48.11 39.68,48.11 38.91,48.87 38.91,50.65 37.64,51.92 J8.4
R0  (via drill 0.41)
  Top 0.203: v36.42,37.49 36.52,37.59 36.52,38.86 U1.P82 | v42.77,39.93 46.33,43.48 46.33,45.41 JP1.5
  Bottom 0.203: v36.42,37.49 38.66,37.49 41.1,39.93 v42.77,39.93
R0_  (via drill 0.41)
  Top 0.203: v77.17,40.79 73.76,37.39 73.25,37.39 72.24,36.37 72.24,35.87 71.63,35.26 70.71,35.26 69.7,36.27 69.7,47.55 J3.5
  Bottom 0.203: R20.1 83.11,42.62 81.28,40.79 v77.17,40.79
R1
  Top 0.203: JP1.7 41.66,45.41 41.66,43.89 40.64,42.88 39.12,42.88 36.07,39.83 36.07,38.91 U1.P83
R1_  (via drill 0.41)
  Top 0.203: v75.03,42.01 74.62,42.01 73.76,42.88 73.25,42.88 72.24,43.89 72.24,45.41 J3.7
  Bottom 0.203: v75.03,42.01 78.64,42.01 79.6,42.98 80.42,42.98 R17.1
R2  (via drill 0.41)
  Top 0.203: v37.8,42.57 35.1,39.88 35.1,38.91 U1.P85
  Bottom 0.203: v37.8,42.57 39.12,43.89 39.12,45.41 JP1.9
R2_
  Bottom 0.203: J3.9 72.24,42.88 74.17,42.88 74.27,42.98 77.78,42.98 R14.1
R-OUT  (via drill 0.41)
  Top 0.203: v6.2,12.6 v7.21,11.58 | v14.78,53.24 v21.23,53.24
  Bottom 0.203: R21.2 2.9,8.59 J4.P$3 2.44,9.14 4.52,11.23 | C4.1 8.18,10.62 v7.21,11.58 | v6.2,12.6 5.89,12.6 4.52,11.23 | v21.23,53.24 22.66,54.66 42.42,54.66 45.11,51.97 45.26,51.97 J8.10 | v14.78,53.24 14.78,52.93 3.71,41.86 3.71,28.19 0.81,25.3 0.81,14.94 4.52,11.23
R_
  Top 0.203: C6.1 80.47,53.8 77.52,53.8 R1.2 77.47,53.7 74.83,53.7 73.76,52.63 73.25,52.63 72.64,52.02 72.64,47.55 J3.8
  Bottom 0.203: R20.2 83.11,44.91 80.52,44.91 R17.2 80.42,44.91 77.78,44.91 R14.2 77.72,44.96 75.23,44.96 J3.8
RIGHT  (via drill 0.41)
  Top 0.203: v27.03,16.05 27.03,17.48 U1.P8
  Bottom 0.203: R21.1 5.64,11.02 9.4,14.78 13.77,14.78 15.09,13.46 23.16,13.46 25.76,16.05 v27.03,16.05
SD_CS  (via drill 0.41)
  Top 0.203: v40.39,37.49 40.08,37.8 40.08,38.86 U1.P75 | v45.62,31.9 v45.62,34.19 | v47.96,29.41 49.89,29.41 49.99,29.52 J2.2
  Bottom 0.203: v40.39,37.49 43.59,37.49 45.62,35.46 v45.62,34.19 | v45.62,31.9 45.62,31.75 v47.96,29.41
SD_MISO  (via drill 0.41)
  Top 0.203: v40.84,28.75 37.14,32.46 37.14,37.9 37.08,37.95 37.08,38.86 U1.P81 | v45.26,25.7 48.01,25.7 49.48,27.18 50.9,27.18 51.56,27.84 51.56,33.93 50.5,35 50.04,35 J2.7
  Bottom 0.203: 43.08,25.7 43.08,26.52 v40.84,28.75 | 43.08,25.7 43.08,24.33 R34.1 | 43.08,25.7 v45.26,25.7
SD_MOSI  (via drill 0.41)
  Top 0.203: v40.69,32.82 39.57,33.93 39.57,38.86 U1.P76 | v47.65,27.74 50.85,27.74 51.16,28.04 51.16,29.97 50.5,30.63 50.04,30.63 J2.3
  Bottom 0.203: v40.69,32.82 45.77,27.74 v47.65,27.74
SD_SCK  (via drill 0.41)
  Top 0.203: v48.06,34.39 49.58,32.87 49.99,32.87 J2.5 | v39.88,40.64 39.07,39.83 39.07,38.91 U1.P77
  Bottom 0.203: v48.06,34.39 48.06,35.66 43.08,40.64 v39.88,40.64
TCK  (via drill 0.41)
  Top 0.203: v17.98,47.45 17.98,45.82 19.2,44.6 19.2,37.59 20.32,36.47 21.59,36.47 U1.P110 | v23.57,53.85 v19,49.28 | v35.97,53.85 37.54,53.85 38.91,52.48 38.91,50.7 40.18,49.43 J8.5
  Bottom 0.203: v17.98,47.45 17.98,48.26 v19,49.28 | v35.97,53.85 v23.57,53.85
TDI  (via drill 0.41)
  Top 0.203: v19.35,18.09 20.68,19.41 21.59,19.41 U1.P144 | v4.52,12.24 4.93,12.24 7.01,10.16 7.57,10.16 17.42,0.3 63.45,0.3 65.58,2.44 65.58,14.73 56.59,23.72 56.59,38.91 53.8,41.71 51.05,41.71 48.87,43.89 48.87,46.94 47.7,48.11 46.53,48.11 45.26,49.38 J8.9
  Bottom 0.203: v19.35,18.09 12.19,18.09 9.3,15.19 7.47,15.19 v4.52,12.24
TDO  (via drill 0.41)
  Top 0.203: v20.12,37.69 20.83,36.98 21.59,36.98 U1.P109 | v17.22,54.66 23.98,54.66 27.89,50.75 27.89,49.63 28.3,49.23 30.58,49.23 34.59,53.24 35.61,53.24 36.37,52.48 v36.37,51
  Bottom 0.203: v20.12,37.69 14.94,37.69 13.36,39.27 13.36,42.93 13.72,43.28 13.72,44.6 12.5,45.82 12.5,49.94 v17.22,54.66 | v36.37,51 36.37,52.48 37.14,53.24 40.69,53.24 41.45,52.48 41.45,50.7 42.72,49.43 J8.7
TMS  (via drill 0.41)
  Top 0.203: v24.94,37.49 24.08,37.49 23.57,38 23.57,38.86 U1.P108 | v28.6,49.94 30.68,49.94 35.41,54.66 44.35,54.66 46.53,52.48 46.53,50.7 47.8,49.43 J8.11
  Bottom 0.203: v24.94,37.49 24.94,44.6 24.89,44.65 24.89,46.23 v28.6,49.94
WR  (via drill 0.41)
  Top 0.203: v18.08,15.95 24.03,15.95 24.54,16.46 24.54,17.48 U1.P3 | v13.82,17.37 11.38,19.81 9.91,19.81 7.11,22.61 4.01,22.61 U3.29
  Bottom 0.203: v18.08,15.95 16.66,17.37 v13.82,17.37
XA0
  Top 0.203: U1.P117 21.59,32.92 16.92,32.92 16.81,32.82 U3.12
XA1
  Top 0.203: U1.P122 21.59,30.48 18.44,30.48 17.42,31.5 16.81,31.5 U3.11
XA2
  Top 0.203: U1.P123 21.59,29.97 17.07,29.97 16.81,30.23 U3.10
XA3
  Top 0.203: U1.P124 21.59,29.41 17.22,29.41 16.81,29.01 U3.9
XA4
  Top 0.203: U1.P125 21.59,28.91 18.59,28.91 17.42,27.74 16.81,27.74 U3.8
XA5
  Top 0.203: U1.P126 21.59,28.45 19.41,28.45 17.42,26.47 16.81,26.47 U3.7
XA6
  Top 0.203: U1.P130 21.59,26.42 19.25,26.42 18.03,25.2 16.81,25.2 U3.6
XA7
  Top 0.203: U1.P131 21.59,25.91 20.12,25.91 18.14,23.93 16.81,23.93 U3.5
XA8  (via drill 0.41)
  Top 0.203: v43.64,42.88 40.59,39.83 40.59,38.91 U1.P74 | v43.64,55.37 10.41,55.37 0.86,45.82 0.86,15.9 v1.52,15.24 | v2.54,16.26 2.54,24.33 3.35,25.15 3.96,25.15 U3.27
  Bottom 0.203: v43.64,42.88 48.26,42.88 48.87,43.48 48.87,46.94 47.7,48.11 47.3,48.11 46.53,48.87 46.53,52.48 v43.64,55.37 | v2.54,16.26 v1.52,15.24
XA9  (via drill 0.41)
  Top 0.203: v20.12,20.47 21.59,20.47 U1.P142 | v8.28,23.06 7.92,23.06 4.57,26.42 4.01,26.42 U3.26
  Bottom 0.203: v20.12,20.47 19.71,20.47 17.12,23.06 v8.28,23.06
XA10
  Top 0.203: U1.P106 24.54,38.91 24.54,39.93 23.47,41 23.47,44.86 20.17,48.16 10.31,48.16 1.83,39.67 1.83,31.8 3.35,30.28 3.96,30.28 U3.23
XA11  (via drill 0.41)
  Top 0.203: v25.25,19.51 23.32,21.44 21.64,21.44 U1.P140 | v13.21,15.95 12.19,15.95 11.12,17.02 11.12,17.63 10.67,18.09 v7.77,18.09 | v2.34,25.81 2.34,26.67 3.35,27.69 3.96,27.69 U3.25
  Bottom 0.203: v25.25,19.51 25.25,18.59 20.68,14.02 15.14,14.02 v13.21,15.95 | v7.77,18.09 2.34,23.52 v2.34,25.81
XA12
  Top 0.203: U1.P132 21.59,25.4 20.22,25.4 17.47,22.66 16.81,22.66 U3.4
XA13  (via drill 0.41)
  Top 0.203: v20.37,18.09 22.1,16.36 23.82,16.36 24.03,16.56 24.03,17.48 U1.P2 | v10.16,20.57 9.75,20.57 6.45,23.88 4.01,23.88 U3.28
  Bottom 0.203: v20.37,18.09 17.88,20.57 v10.16,20.57
XA14
  Top 0.203: U1.P134 21.59,24.43 20.17,24.43 18.24,22.5 18.24,22.2 17.42,21.39 16.81,21.39 U3.3
XA15  (via drill 0.41)
  Top 0.203: v16.36,16.66 18.59,14.43 23.42,14.43 25.55,16.56 25.55,17.48 U1.P5 | v12.5,16.66 12.5,17.07 11.94,17.63 11.94,18.03 10.97,19 9.5,19 6.71,21.79 6.1,21.79 5.38,21.08 5.38,20.93 4.57,20.12 4.01,20.12 U3.31
  Bottom 0.203: v12.5,16.66 v16.36,16.66
XA16  (via drill 0.41)
  Top 0.203: v24.99,25.6 23.37,23.98 21.64,23.98 U1.P135 | v26.42,25.65 26.42,19.76 v26.16,19.51 | v19.81,15.24 v22.91,15.24 | v17.68,17.37 16.41,17.37 15.39,18.39 15.39,19.25 16.2,20.07 16.76,20.07 U3.2
  Bottom 0.203: v24.99,25.6 26.36,25.6 v26.42,25.65 | v26.16,19.51 26.16,18.49 v22.91,15.24 | v17.68,17.37 v19.81,15.24
XA17
  Top 0.203: U1.P139 21.59,21.95 20.73,21.95 19.96,21.18 19.76,21.18 17.42,18.85 16.81,18.85 U3.1
XA18  (via drill 0.41)
  Top 0.203: v24.54,18.9 25.04,18.39 25.04,17.53 U1.P4 | v14.22,15.95 12.35,17.83 12.35,18.24 11.18,19.41 9.7,19.41 6.91,22.2 5.38,22.2 4.57,21.39 4.01,21.39 U3.30
  Bottom 0.203: v24.54,18.9 24.54,18.75 20.22,14.43 15.75,14.43 v14.22,15.95
XD0
  Top 0.203: U1.P116 21.59,33.48 17.37,33.48 16.81,34.04 U3.13
XD1
  Top 0.203: U1.P113 21.59,34.95 20.68,34.95 20.32,35.31 16.81,35.31 U3.14
XD2  (via drill 0.41)
  Top 0.203: v22.76,39.32 22.76,35.71 22.5,35.46 21.64,35.46 U1.P112 | v18.24,38.96 18.24,37.44 17.42,36.63 16.81,36.63 U3.15
  Bottom 0.203: v22.76,39.32 20.98,41.1 20.37,41.1 v18.24,38.96
XD3  (via drill 0.41)
  Top 0.203: v20.47,49.68 29.06,41.1 29.06,38.91 U1.P97 | v17.37,50.39 11.53,50.39 v3,41.86 | v3,38.81 3.96,37.85 U3.17
  Bottom 0.203: v20.47,49.68 20.22,49.68 19.51,50.39 v17.37,50.39 | v3,38.81 v3,41.86
XD4  (via drill 0.41)
  Top 0.203: v27.63,32.77 28.7,33.83 28.7,37.64 28.6,37.74 28.6,38.86 U1.P98 | v5.59,35.97 4.62,35.97 4.01,36.58 U3.18
  Bottom 0.203: v27.63,32.77 27.63,32.36 26.26,30.99 10.21,30.99 5.59,35.61 v5.59,35.97
XD5  (via drill 0.41)
  Top 0.203: v11.73,48.87 12.04,48.56 20.98,48.56 26.06,43.48 26.06,38.91 U1.P103 | v4.42,41.25 2.29,39.12 2.29,36.42 3.35,35.36 3.96,35.36 U3.19
  Bottom 0.203: v11.73,48.87 4.42,41.55 v4.42,41.25
XD6  (via drill 0.41)
  Top 0.203: v24.18,44.35 25.55,42.98 25.55,38.91 U1.P104 | v14.94,47.45 14.53,47.45 14.33,47.65 10.52,47.65 6.86,43.99 6.86,36.22 4.73,34.09 4.01,34.09 U3.20
  Bottom 0.203: v24.18,44.35 24.18,44.96 19.71,49.43 19.71,49.58 19.3,49.99 18.19,49.99 15.65,47.45 v14.94,47.45
XD7  (via drill 0.41)
  Top 0.203: v24.18,43.13 24.18,40.89 25.04,40.03 25.04,38.91 U1.P105 | v22.76,44.55 22.76,42.67 v21.59,41.5 | v14.07,39.57 7.32,32.82 4.01,32.82 U3.21
  Bottom 0.203: v22.76,44.55 v24.18,43.13 | v21.59,41.5 16.2,41.5 14.28,39.57 v14.07,39.57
